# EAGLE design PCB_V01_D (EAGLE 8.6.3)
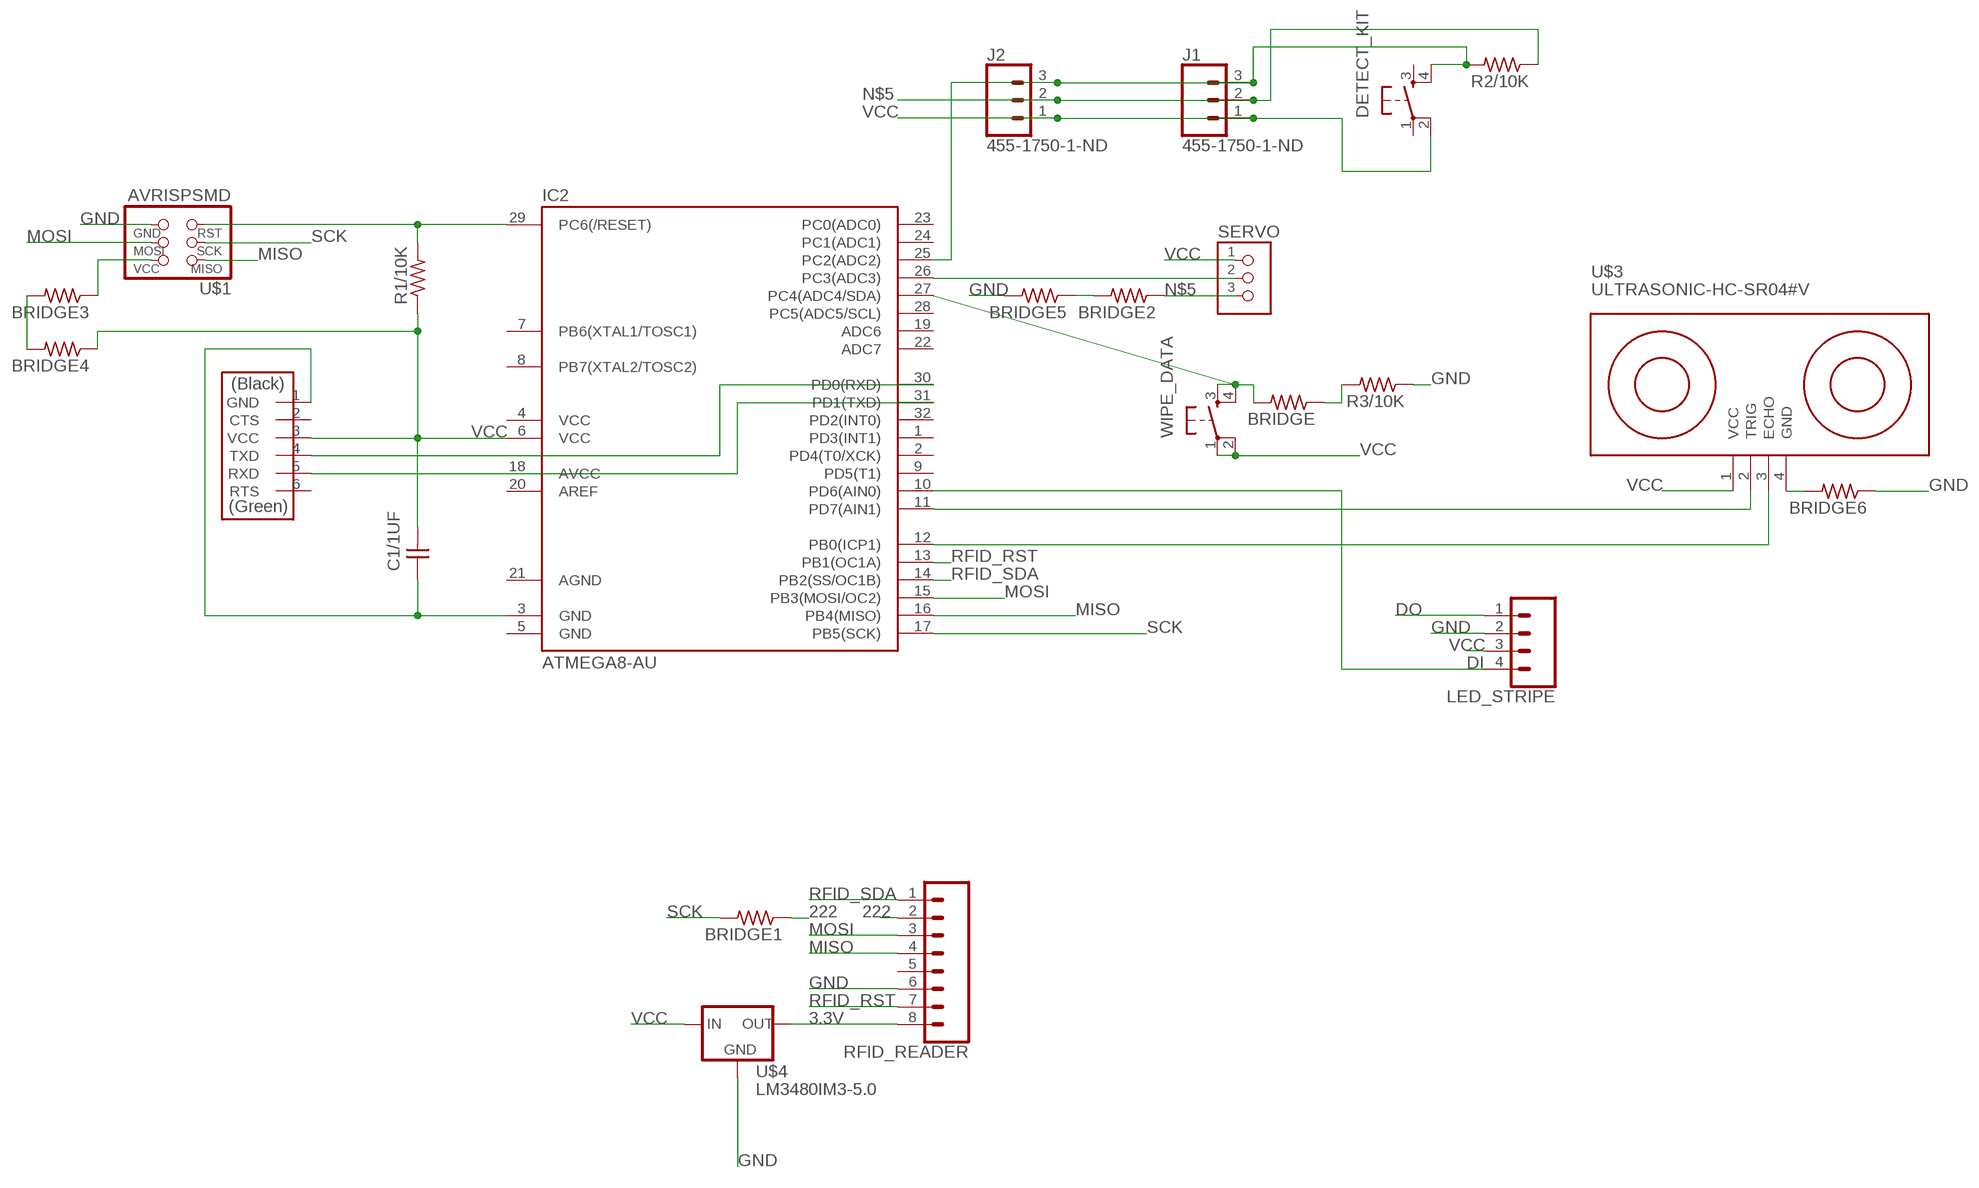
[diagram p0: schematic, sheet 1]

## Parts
BRIDGE  RES-US1206FAB  [R1206FAB]
BRIDGE1  RES-US1206FAB  [R1206FAB]
BRIDGE2  RES-US1206FAB  [R1206FAB]
BRIDGE3  RES-US1206FAB  [R1206FAB]
BRIDGE4  RES-US1206FAB  [R1206FAB]
BRIDGE5  RES-US1206FAB  [R1206FAB]
BRIDGE6  RES-US1206FAB  [R1206FAB]
C1/1UF  CAP-UNPOLARIZEDFAB  [C1206FAB]
DETECT_KIT  6MM_SWITCH6MM_SWITCH  [6MM_SWITCH]
IC2  ATMEGA8-AU  [TQFP32-08]
J1  455-1750-1-ND  CONN_03  [1X03]
J2  455-1750-1-ND  CONN_03  [1X03]
LED_STRIPE  CONN_04  [1X04]
R1/10K  RES-US1206FAB  [R1206FAB]
R2/10K  RES-US1206FAB  [R1206FAB]
R3/10K  RES-US1206FAB  [R1206FAB]
RFID_READER  CONN_08"  [1X08]
SERVO  TERM-1X03'-FABLAB'  [ED555DS-3DS]
U$1  AVRISPSMD  [2X03SMD]
U$2  FTDI-SMD-HEADER  [1X06SMD]
U$3  ULTRASONIC-HC-SR04#V  [ULTRASONIC-HC-SR04#V]
U$4  LM3480IM3-5.0  [SOT23]
WIPE_DATA  6MM_SWITCH6MM_SWITCH  [6MM_SWITCH]

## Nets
3.3V: RFID_READER.8 U$4.1(OUT)
222: BRIDGE1.1 RFID_READER.2
DI: IC2.10(PD6(AIN0)) LED_STRIPE.4
DO: LED_STRIPE.1
GND: BRIDGE2.2 BRIDGE5.1 BRIDGE5.2 BRIDGE6.1 C1/1UF.1 IC2.3(GND) LED_STRIPE.2 R3/10K.1 RFID_READER.6 U$1.6(GND) U$2.1(GND) U$4.3(GND)
MISO: IC2.16(PB4(MISO)) RFID_READER.4 U$1.1(MISO)
MOSI: IC2.15(PB3(MOSI/OC2)) RFID_READER.3 U$1.4(MOSI)
N$1: IC2.11(PD7(AIN1)) U$3.2(TRIG)
N$2: BRIDGE.1 R3/10K.2
N$3: IC2.29(PC6(/RESET)) R1/10K.2 U$1.5(RST)
N$4: IC2.26(PC3(ADC3)) SERVO.2
N$5: BRIDGE2.1 J1.2 J2.2 R2/10K.1 SERVO.3
N$6: BRIDGE.2 IC2.27(PC4(ADC4/SDA)) WIPE_DATA.3(S) WIPE_DATA.4(S1)
N$7: IC2.12(PB0(ICP1)) U$3.3(ECHO)
N$8: IC2.31(PD1(TXD)) U$2.5(RXD)
N$9: IC2.30(PD0(RXD)) U$2.4(TXD)
N$10: DETECT_KIT.4(S1) IC2.25(PC2(ADC2)) J1.3 J2.3 R2/10K.2
N$11: BRIDGE3.2 BRIDGE4.2
N$12: BRIDGE6.2 U$3.4(GND)
N$13: BRIDGE3.1 U$1.2(VCC)
RFID_RST: IC2.13(PB1(OC1A)) RFID_READER.7
RFID_SDA: IC2.14(PB2(SS/OC1B)) RFID_READER.1
SCK: BRIDGE1.2 IC2.17(PB5(SCK)) U$1.3(SCK)
VCC: BRIDGE4.1 C1/1UF.2 DETECT_KIT.2(P1) IC2.6(VCC) J1.1 J2.1 LED_STRIPE.3 R1/10K.1 SERVO.1 U$2.3(VCC) U$3.1(VCC) U$4.2(IN) WIPE_DATA.1(P) WIPE_DATA.2(P1)
Unconnected: DETECT_KIT.1(P) DETECT_KIT.3(S) IC2.1(PD3(INT1)) IC2.2(PD4(T0/XCK)) IC2.7(PB6(XTAL1/TOSC1)) IC2.8(PB7(XTAL2/TOSC2)) IC2.9(PD5(T1)) IC2.18(AVCC) IC2.19(ADC6) IC2.20(AREF) IC2.22(ADC7) IC2.23(PC0(ADC0)) IC2.24(PC1(ADC1)) IC2.28(PC5(ADC5/SCL)) IC2.32(PD2(INT0)) RFID_READER.5 U$2.2(CTS) U$2.6(RTS)

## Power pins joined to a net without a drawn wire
AGND: IC2.21(AGND)
GND: IC2.5(GND)
VCC: IC2.4(VCC)

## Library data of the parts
BRIDGE BRIDGE1-BRIDGE6 R1/10K R2/10K R3/10K = fab:RES-US: Resistor (US Symbol)
C1/1UF = fab:CAP-UNPOLARIZED
DETECT_KIT WIPE_DATA = fab:6MM_SWITCH: OMRON SWITCH
IC2 = atmega8:ATMEGA8
J1 J2 = SparkFun-Connectors:CONN_03: Multi connection point. Often used as Generic Header-pin footprint for 0.1 inch spaced/style header connections On any of the 0.1 inch spaced packages, you can populate with these: Break Away Headers - Straight (PRT-00116) Break Away Male Headers - Right Angle (PRT-00553) Female Headers (PRT-00115)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; PROD_ID: XXX-00000
LED_STRIPE = SparkFun-Connectors:CONN_04: Multi connection point. Often used as Generic Header-pin footprint for 0.1 inch spaced/style header connections On any of the 0.1 inch spaced packages, you can populate with these: Break Away Headers - Straight (PRT-00116) Break Away Male Headers - Right Angle (PRT-00553) Female Headers (PRT-00115)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; PROD_ID: CONN-09696
RFID_READER = SparkFun-Connectors:CONN_08: Multi connection point. Often used as Generic Header-pin footprint for 0.1 inch spaced/style header connections On any of the 0.1 inch spaced packages, you can populate with these: Break Away Headers - Straight (PRT-00116) Break Away Male Headers - Right Angle (PRT-00553) Female Headers (PRT-00115)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; PROD_ID: CONN-08438
SERVO = fab:TERM-1X03: 3.5mm terminal block, 3 positions ED555-3DS as found in the fablab inventory. Made by Zaerc.
U$1 = fab:AVRISP
U$2 = fab:FTDI-SMD-HEADER
U$3 = diy-modules:ULTRASONIC-HC-SR04: Ultrasonic Ranging Module HC-SR04 More details available here: http://randomnerdtutorials.com/complete-guide-for-ultrasonic-sensor-hc-sr04/ Click here to find device on ebay.com
U$4 = national_gaui:LM3480

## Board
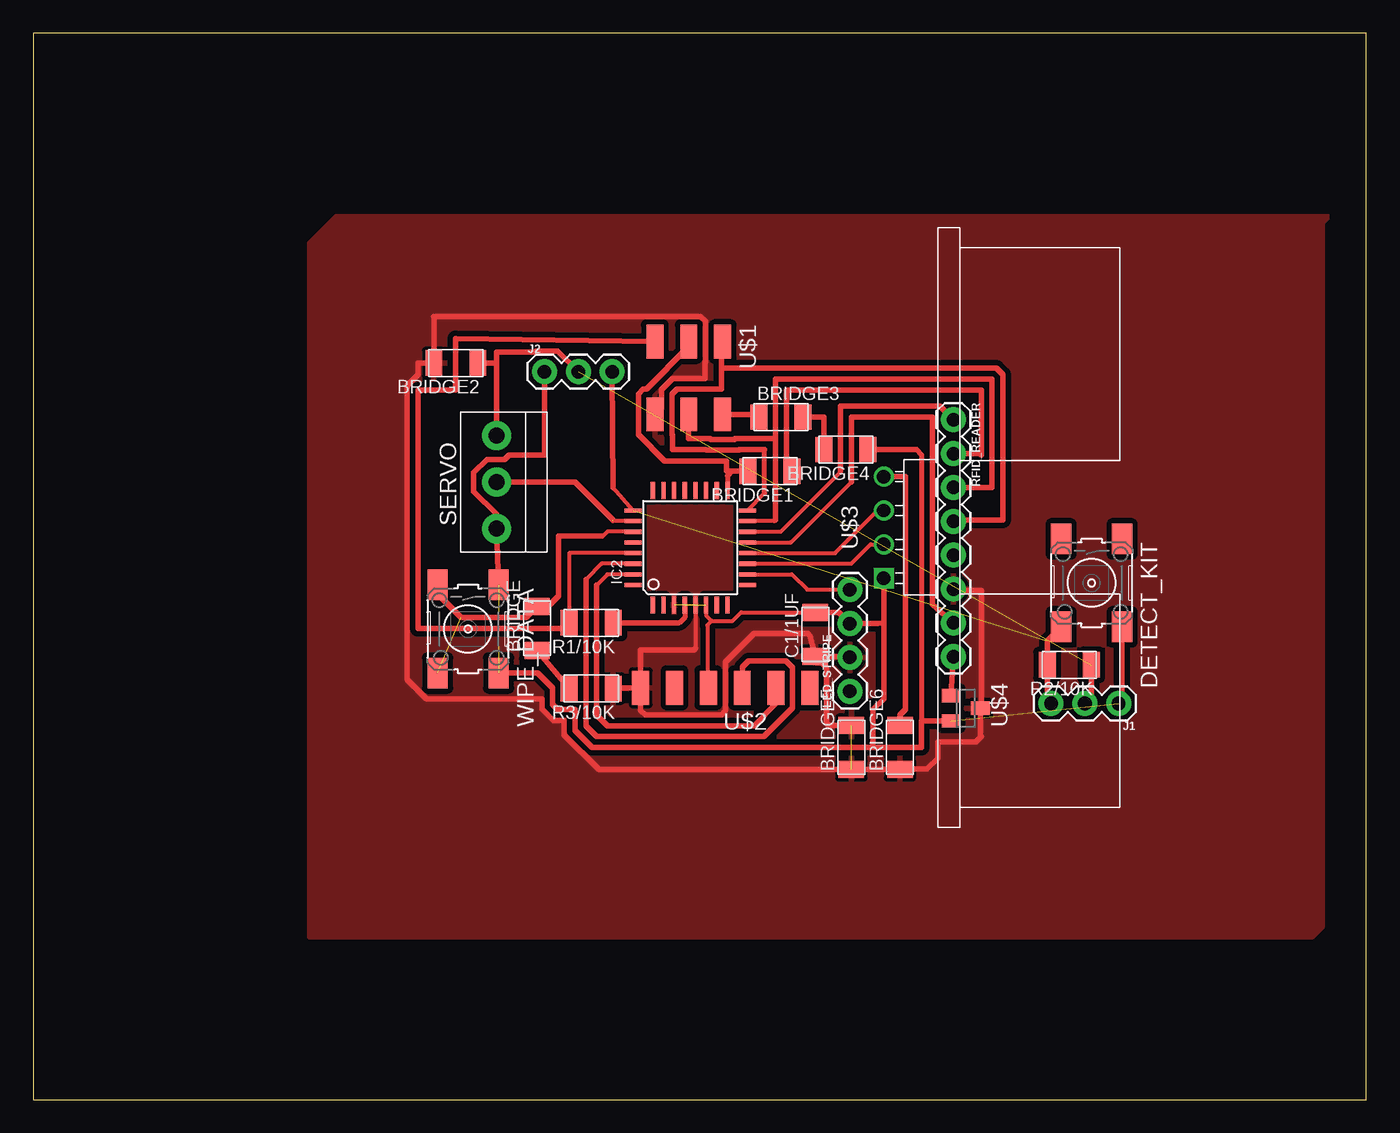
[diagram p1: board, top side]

Size 100 x 80 mm. Coordinates in mm from the lower left corner, seen from the top.
Outline: 0,0 100,0 100,80 0,80 0,0
Copper layers (1*16): Top 0.035mm / dielectric 1.5mm / Bottom 0.035mm
Design rules "default *": minimum track width 6mil, minimum drill 0.35mm, track to track 16mil, track to pad 16mil, pad to pad 16mil, via to via 16mil, smd to smd 16mil, copper to edge 40mil, drill to drill 6mil, minimum pad ring 10mil, minimum via ring 8mil, stop-mask expansion 4mil, vias tented up to drill 0mil, thermal gap 10mil

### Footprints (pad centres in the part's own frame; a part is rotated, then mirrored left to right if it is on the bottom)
R1206FAB = smd 1.27 x 1.905: 1 -1.651,0; 2 1.651,0
C1206FAB = smd 1.27 x 1.905: 1 -1.651,0; 2 1.651,0
6MM_SWITCH = smd 2.286 x 1.524: 1 -3.302,2.286; 2 3.302,2.286; 3 -3.302,-2.286; 4 3.302,-2.286
TQFP32-08 = smd 1.27 x 0.305: 1 -4.293,2.8; 2 -4.293,2; 3 -4.293,1.2; 4 -4.293,0.4; 5 -4.293,-0.4; 6 -4.293,-1.2; 7 -4.293,-2; 8 -4.293,-2.8; 17 4.293,-2.8; 18 4.293,-2; 19 4.293,-1.2; 20 4.293,-0.4; 21 4.293,0.4; 22 4.293,1.2; 23 4.293,2; 24 4.293,2.8 | smd 0.305 x 1.27: 9 -2.8,-4.293; 10 -2,-4.293; 11 -1.2,-4.293; 12 -0.4,-4.293; 13 0.4,-4.293; 14 1.2,-4.293; 15 2,-4.293; 16 2.8,-4.293; 25 2.8,4.293; 26 2,4.293; 27 1.2,4.293; 28 0.4,4.293; 29 -0.4,4.293; 30 -1.2,4.293; 31 -2,4.293; 32 -2.8,4.293
1X03 = drill 1.016 pad 1.88: 1 0,0; 2 2.54,0; 3 5.08,0
1X04 = drill 1.016 pad 1.88: 1 0,0; 2 2.54,0; 3 5.08,0; 4 7.62,0
1X08 = drill 1.016 pad 1.88: 1 0,0; 2 2.54,0; 3 5.08,0; 4 7.62,0; 5 10.16,0; 6 12.7,0; 7 15.24,0; 8 17.78,0
ED555DS-3DS = drill 1.2 pad 2.184: 1 -3.5,0; 2 0,0; 3 3.5,0
2X03SMD = smd 2.54 x 1.27: 1 -2.54,2.54; 2 2.92,2.54; 3 -2.54,0; 4 2.92,0; 5 -2.54,-2.54; 6 2.92,-2.54
1X06SMD = smd 2.54 x 1.27: 1 0,6.35; 2 0,3.81; 3 0,1.27; 4 0,-1.27; 5 0,-3.81; 6 0,-6.35
ULTRASONIC-HC-SR04#V = drill 1 square: 1 -3.81,0 | drill 1: 2 -1.27,0; 3 1.27,0; 4 3.81,0
SOT23 = smd 1 x 1.4: 1 -0.95,-1.1; 2 0.95,-1.1; 3 0,1.1

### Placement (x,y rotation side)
BRIDGE  37.8,35.36 90 top
BRIDGE1  55.27,47.14 180 top
BRIDGE2  31.7,55.27 180 top
BRIDGE3  56.08,51.21 0 top
BRIDGE4  60.96,48.77 180 top
BRIDGE5  61.37,26.42 90 top
BRIDGE6  65.02,26.42 90 top
C1/1UF  58.67,34.9 90 top
DETECT_KIT  79.4,38.76 270 top
IC2  49.28,41.4 90 top
J1  81.43,29.72 180 top
J2  38.35,54.61 0 top
LED_STRIPE  61.26,30.63 90 top
R1/10K  41.86,35.76 180 top
R2/10K  77.72,32.61 180 top
R3/10K  41.86,30.84 180 top
RFID_READER  69.04,51 270 top
SERVO  34.75,46.33 90 top
U$1  49.17,54.33 270 top
U$2  51.92,30.89 90 top
U$3  63.8,42.93 90 top
U$4  69.95,29.36 270 top
WIPE_DATA  32.61,35.31 270 top

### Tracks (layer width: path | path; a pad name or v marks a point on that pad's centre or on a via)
3.3V
  Top 0.406: U$4.1 RFID_READER.8
222
  Top 0.406: RFID_READER.2 71.02,48.46 71.12,48.36 71.12,53.24 56.49,53.24 56.49,47.57 BRIDGE1.1
DI
  Top 0.305: IC2.10 56.91,39.4 58.06,38.25 LED_STRIPE.4
GND  (2 unrouted)
  Top 0.305: IC2.5 49.68,33.83
  Top 0.406: U$1.6 47.12,51.89 47.12,53.27 47.95,54.1 50.39,54.1 50.39,55.32 50.42,55.35 50.42,58.39 50.06,58.75 30.07,58.75 | R3/10K.1 43.51,30.89 U$2.1 | U$2.1 45.57,33.73 49.58,33.73 49.68,33.83 | 30.05,58.75 30.07,58.75 | RFID_READER.6 69.14,38.2 71.12,38.2 71.12,29.43 U$4.3 71.05,27.3 71.12,27.23 70.71,26.82 67.87,26.82 67.87,25.6 67.06,24.79 65.05,24.79 BRIDGE6.1 BRIDGE5.1 42.43,24.77 39.83,27.37 39.83,28.45 39,28.45 38.15,29.29 38.15,30.07 29.49,30.07 28.04,31.52 28.04,53.58 28.85,54.39 28.85,55.27 BRIDGE2.2 30.07,55.3 30.07,58.75 | C1/1UF.1 61.19,33.25 LED_STRIPE.2 | C1/1UF.1 58.75,32.77 59.16,32.77 59.51,32.41 59.51,28.27 59.74,28.04 59.77,28.07 BRIDGE5.2 | U$2.1 45.57,29.21 45.92,28.85 51.61,28.85 51.94,29.18 51.94,32.84 54.05,34.95 58.12,34.95 58.27,34.8 C1/1UF.1
  pour Top: 20.73,64.21 20.73,12.19 95.91,12.19 96.72,13 96.72,65.84 97.13,66.24 22.76,66.24
MISO
  Top 0.305: IC2.16 54.86,45.5
  Top 0.381: 54.86,45.5 54.86,48.77
  Top 0.406: U$1.1 51.61,56.77 51.61,54.86 | 51.61,54.86 51.61,53.29 48.29,53.29 47.93,52.93 47.93,49.89 47.95,49.86 47.95,48.77 50.44,48.77 50.49,48.72 52.94,48.72 52.99,48.77 54.86,48.77 | RFID_READER.4 69.14,43.48 72.75,43.48 72.75,54.39 72.27,54.86 51.61,54.86
MOSI
  Top 0.305: 55.68,43.48 55.59,43.4 IC2.15
  Top 0.406: 55.68,49.58 55.68,43.48 | U$1.4 49.17,49.58 50.78,49.58 50.83,49.53 52.6,49.53 52.65,49.58 55.68,49.58 | RFID_READER.3 71.93,45.92 71.93,54.05 55.68,54.05 55.68,49.58
N$1
  Top 0.305: IC2.11 61.37,40.2 62.82,41.66 U$3.2
N$2
  Top 0.406: R3/10K.2 BRIDGE.1
N$3
  Top 0.305: IC2.29 40.21,41 R1/10K.2
  Top 0.406: U$1.5 31.7,57.1 31.7,53.24 28.85,53.24 28.85,35.36 39.8,35.36 R1/10K.2
N$4  (1 unrouted)
  Top 0.305: IC2.26 43.48,43.4
  Top 0.406: 43.48,43.48 40.64,46.33 SERVO.2
N$5  (1 unrouted)
  Top 0.406: SERVO.3 34.75,55.27 | 34.75,55.27 BRIDGE2.1 | J2.2 39.34,56.16 37.71,56.16 37.64,56.08 34.75,56.08 34.75,55.27 | R2/10K.1 79.38,30.2 J1.2
N$6  (1 unrouted)
  Top 0.305: IC2.27 43.08,42.6 42.74,42.27 42.67,42.27
  Top 0.406: WIPE_DATA.3 30.33,37.95 32.11,36.17 36.96,36.17 BRIDGE.2 38.61,37.01 39.4,37.8 39.4,41.86 39.42,42.27 42.67,42.27
N$7
  Top 0.305: IC2.12 60.15,41 63.2,44.05 63.68,44.05
  Top 0.406: 63.68,44.05 U$3.3
N$8
  Top 0.305: IC2.31 43.08,39.4 42.28,38.61
  Top 0.381: 42.28,38.61 42.27,38.61
  Top 0.406: 42.27,38.61 42.27,28.85 43.08,28.04 54.05,28.04 55.73,29.72 U$2.5 55.73,31.65 55.68,31.7
N$9
  Top 0.305: IC2.30 42.64,40.2 41.45,39.01
  Top 0.406: 41.45,39.01 41.45,28.04 42.27,27.23 54.84,27.23 56.97,29.36 56.97,32.41 56.46,32.92 53.65,32.92 53.19,32.46 U$2.4
N$10  (1 unrouted)
  Top 0.305: IC2.25 43.48,45.92
  Top 0.406: 43.48,45.92 J2.3 | J1.3 76.07,30 R2/10K.2 76.07,34.42 DETECT_KIT.4
N$11
  Top 0.406: BRIDGE3.2 59.33,51.21 59.31,51.18 BRIDGE4.2
N$12
  Top 0.406: BRIDGE6.2 65.02,28.85 65.43,29.26 65.43,46.74 U$3.4
N$13
  Top 0.406: U$1.2 54.23,51.41 BRIDGE3.1
RFID_RST
  Top 0.305: IC2.13 56.84,41.8 61.37,46.33
  Top 0.406: RFID_READER.7 67.44,37.16 67.46,49.58 67.46,51.21 61.37,51.21 61.37,46.33
RFID_SDA
  Top 0.305: IC2.14 56.08,42.6 60.55,47.07
  Top 0.381: 60.55,47.07 60.55,47.14
  Top 0.406: 60.55,47.14 60.55,52.02 68.02,52.02 RFID_READER.1
SCK
  Top 0.381: 52.43,47.14 52.08,46.79 IC2.17
  Top 0.406: U$1.3 49.17,56.48 45.99,53.29 45.75,53.29 45.39,52.93 45.39,49.89 47.37,47.9 52.02,47.9 52.02,47.14 52.43,47.14 BRIDGE1.2
VCC  (3 unrouted)
  Top 0.305: IC2.6 50.48,36.33 50.89,35.92 | C1/1UF.2 53.09,36.55 52.46,35.92 50.89,35.92 | 50.89,35.92 50.57,35.59 50.57,30.89
  Top 0.381: IC2.4 48.88,36.17 48.47,35.76 48.36,35.76 | 66.24,48.77 66.65,48.36 66.65,41.78 66.64,37.46 66.62,37.43 66.64,37.13 66.64,36.83 66.65,36.82 66.65,28.41
  Top 0.406: WIPE_DATA.1 SERVO.1 34.75,43.92 33.05,45.62 33.05,47.03 34.04,48.03 35.36,48.03 35.69,48.36 38.35,48.36 J2.1 | 50.57,30.89 U$2.3 | 48.36,35.76 R1/10K.1 | U$3.1 63.8,35.76 | 63.8,35.76 63.8,30.07 62.99,29.26 62.99,26.42 | U$4.2 66.65,28.41 | 63.8,35.76 63.35,35.71 LED_STRIPE.3 60.43,36.55 C1/1UF.2 | BRIDGE4.1 65.83,48.77 66.24,48.77 | 66.65,28.41 | WIPE_DATA.2 37.85,32 38.96,30.89 38.96,29.63 39.33,29.26 40.64,29.26 40.64,27.7 41.93,26.42 62.99,26.42 | 62.99,26.42 66.65,26.42 66.65,28.41 | DETECT_KIT.2 81.69,29.97 J1.1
